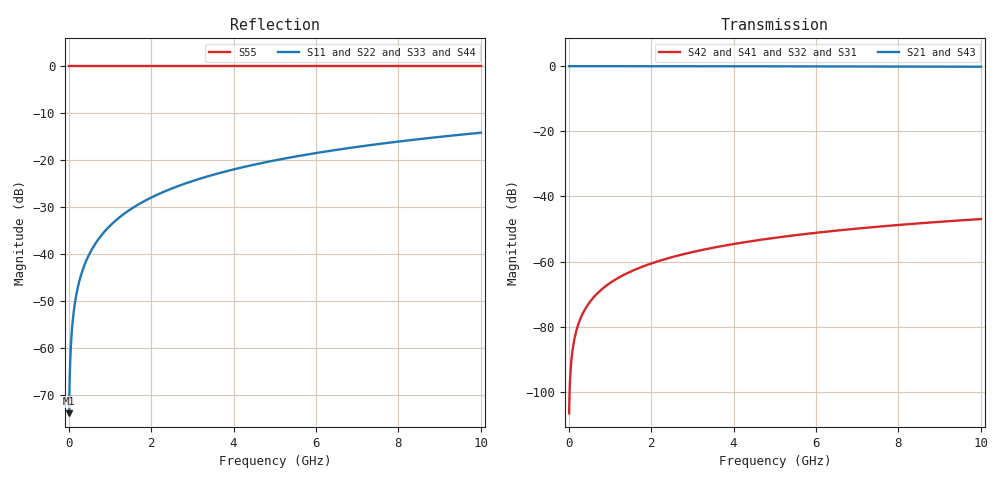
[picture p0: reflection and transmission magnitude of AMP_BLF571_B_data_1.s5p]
! Created Tue Sep 29 12:15:48 2009
# ghz S ma R 50
! 5 Port Network Data from SP1.SP block
! freq  magS11  angS11  magS12  angS12  magS13  angS13  magS14  angS14
!  magS15  angS15
!  magS21  angS21  magS22  angS22  magS23  angS23
!  magS24  angS24  magS25  angS25
!  magS31  angS31  magS32  angS32
!  magS33  angS33  magS34  angS34  magS35  angS35
!  magS41  angS41
!  magS42  angS42  magS43  angS43  magS44  angS44  magS45  angS45
!  magS51  angS51  magS52  angS52  magS53  angS53  magS54  angS54
!  magS55  angS55
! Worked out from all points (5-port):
!   1000 points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, 10 MHz to 10 GHz, reference 50 ohm
!   strongest paths, dB at 10 MHz, 2.51 GHz, 5.01 GHz, 7.51 GHz, 10 GHz:
!     S21: 0.0, 0.0, 0.0, -0.1, -0.2
!     S43: 0.0, 0.0, 0.0, -0.1, -0.2
!     S42: -106.6, -58.6, -52.7, -49.3, -46.9
!     S41: -106.6, -58.6, -52.7, -49.3, -46.9
!     S32: -106.6, -58.6, -52.7, -49.3, -46.9
!     S31: -106.6, -58.6, -52.7, -49.3, -46.9
!   lowest |S11| = -73.9 dB at 10 MHz (marker M1), VSWR 1.00, Z = 50 + j0.02 ohm
!   |S11| at or under -10 dB: start of sweep to end of sweep
